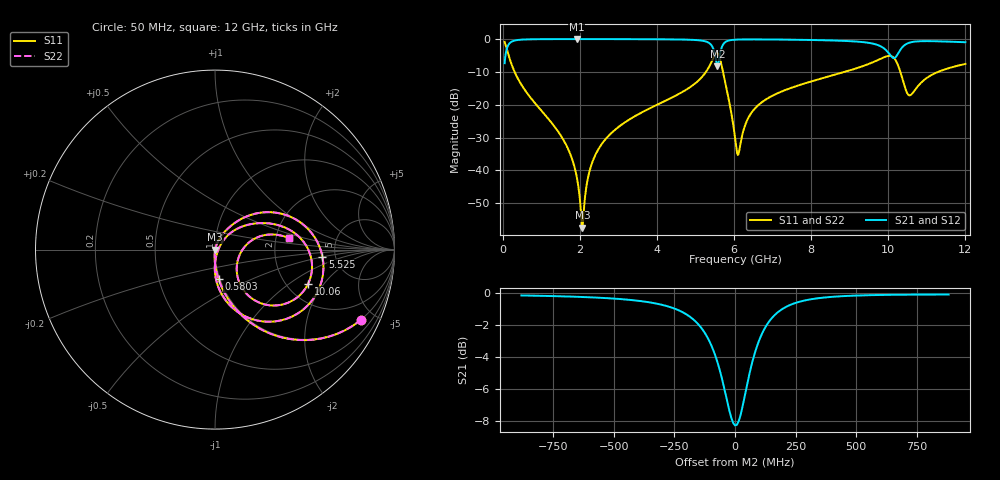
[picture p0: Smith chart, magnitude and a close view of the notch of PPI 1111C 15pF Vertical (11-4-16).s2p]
# GHz S MA R 50
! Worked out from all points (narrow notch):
!   1601 points, 50 MHz to 12 GHz, reference 50 ohm
!   highest |S21| = -0.01 dB at 1.925 GHz (marker M1); lowest = -8.3 dB at 5.569 GHz (marker M2)
!   notch at M2: 8.1 dB deep, 147 MHz wide at half that depth
!   lowest |S11| = -57.4 dB at 2.067 GHz (marker M3), VSWR 1.00, Z = 50.1 - j0.0168 ohm
!   |S11| at or under -10 dB: 309.6 MHz to 5.272 GHz (4.962 GHz wide, 178 % of centre); 5.714 GHz to 8.87 GHz (3.156 GHz wide, 43.3 % of centre); 10.31 GHz to 11.29 GHz (980.7 MHz wide, 9.08 % of centre)
!   |S22| runs from -57.4 to -0.9 dB; largest |S21 - S12| = 0
!   S11 on the Smith chart (normalised r, x): 50 MHz: 0.98, -4.18; 580.3 MHz: 0.98, -0.33; 5.525 GHz: 3.94, -0.48; 10.06 GHz: 2.58, -1.43; 12 GHz: 2.37, +0.37
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0.05  0.9035 -25.6  0.4285 64.4  0.4285 64.4  0.9035 -25.6
0.2367188  0.4026 -67.4  0.9149 22.6  0.9149 22.6  0.4026 -67.4
0.5802812  0.1659 -83.1  0.9854 6.7  0.9854 6.7  0.1659 -83.1
1.558688  0.03028 -93.8  0.9983 -6.0  0.9983 -6.0  0.03028 -93.8
1.924656  0.00776 -89.5  0.9986 -9.1  0.9986 -9.1  0.00776 -89.5
2.044156  0.001741 -50.1  0.9985 -10.1  0.9985 -10.1  0.001741 -50.1
2.066562  0.001343 -7.1  0.9985 -10.2  0.9985 -10.2  0.001343 -7.1
2.268219  0.01054 70.5  0.9984 -11.8  0.9984 -11.8  0.01054 70.5
2.5595  0.0247 72.4  0.998 -14.1  0.998 -14.1  0.0247 72.4
4.038312  0.1021 62.9  0.9919 -25.6  0.9919 -25.6  0.1021 62.9
5.121281  0.2472 47.2  0.9532 -39.2  0.9532 -39.2  0.2472 47.2
5.524594  0.5999 -3.7  0.5059 -54.5  0.5059 -54.5  0.5999 -3.7
5.569406  0.6171 -23.3  0.3859 -32.9  0.3859 -32.9  0.6171 -23.3
5.741187  0.2656 -80.3  0.8638 -13.7  0.8638 -13.7  0.2656 -80.3
6.025  0.03173 -75.0  0.9778 -27.8  0.9778 -27.8  0.03173 -75.0
6.122094  0.01836 -1.0  0.9836 -30.1  0.9836 -30.1  0.01836 -1.0
6.734531  0.1107 47.8  0.9868 -38.7  0.9868 -38.7  0.1107 47.8
8.019156  0.2277 37.2  0.9672 -51.2  0.9672 -51.2  0.2277 37.2
10.01331  0.5539 -14.4  0.6067 -75.6  0.6067 -75.6  0.5539 -14.4
10.05813  0.5526 -20.3  0.5615 -72.7  0.5615 -72.7  0.5526 -20.3
10.55106  0.1388 -19.2  0.8814 -53.2  0.8814 -53.2  0.1388 -19.2
12  0.418 8.8  0.8936 -79.2  0.8936 -79.2  0.418 8.8
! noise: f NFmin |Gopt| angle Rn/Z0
0.05  0.0003734  0.8692  1.464  0.0006144
1.372  0.003793  0.6769  7  0.002258
2.701  0.006437  0.6371  13.15  0.003302
4.031  0.01004  0.6539  19.22  0.005375
5.36  0.05759  0.9091  25.92  0.1323
6.682  0.02052  0.7198  31.78  0.01344
8.012  0.02107  0.6877  37.08  0.01183
9.341  0.04492  0.8211  43.27  0.04556
10.67  0.0855  0.8918  49.19  0.1424
12  0.03888  0.7604  53.5  0.02635
